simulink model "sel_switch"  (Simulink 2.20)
settings: Solver=ode45  StartTime=0.0  StopTime=10.0  RelTol=1e-3  AbsTol=1e-6

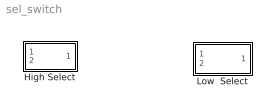
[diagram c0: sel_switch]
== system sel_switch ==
  High Select : Subsystem
  Low  Select : Subsystem

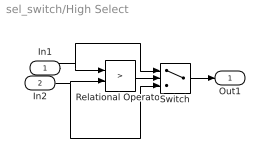
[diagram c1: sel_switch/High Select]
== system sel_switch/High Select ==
  In1 : Inport  Port=1  PortWidth=-1  SampleTime=-1
  In2 : Inport  Port=2  PortWidth=-1  SampleTime=-1
  Relational Operator : RelationalOperator  Operator=>
  Switch : Switch  Threshold=.5
  Out1 : Outport  Port=1  InitialOutput=0
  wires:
  Relational Operator/1 -> Switch/2
  In2/1 -> Relational Operator/2, Switch/3
  In1/1 -> Relational Operator/1, Switch/1
  Switch/1 -> Out1/1

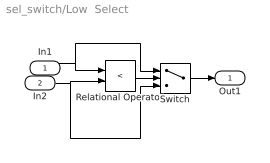
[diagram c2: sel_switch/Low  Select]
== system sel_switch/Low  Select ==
  In1 : Inport  Port=1  PortWidth=-1  SampleTime=-1
  In2 : Inport  Port=2  PortWidth=-1  SampleTime=-1
  Relational Operator : RelationalOperator  Operator=<
  Switch : Switch  Threshold=.5
  Out1 : Outport  Port=1  InitialOutput=0
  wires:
  Switch/1 -> Out1/1
  In1/1 -> Switch/1, Relational Operator/1
  In2/1 -> Switch/3, Relational Operator/2
  Relational Operator/1 -> Switch/2
